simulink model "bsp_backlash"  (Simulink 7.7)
settings: Solver=ode45  StartTime=0.0  StopTime=10.0  MaxStep=0.1  RelTol=1e-3
StopFcn:
  | bsp_backlash_plot

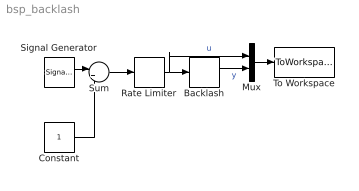
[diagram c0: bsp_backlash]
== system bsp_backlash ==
  Backlash : Backlash
  Constant : Constant
  Mux : Mux  Inputs=2
  Rate Limiter : RateLimiter
  Signal Generator : SignalGenerator  WaveForm=square  Frequency=0.4
  Sum : Sum  Inputs=|++
  To Workspace : ToWorkspace  VariableName=ausgabe  SampleTime=-1  SaveFormat=Array
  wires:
  Constant/1 -> Sum/2
  Signal Generator/1 -> Sum/1
  Rate Limiter/1 -> Backlash/1, Mux/1  "u"
  Mux/1 -> To Workspace/1
  Backlash/1 -> Mux/2  "y"
  Sum/1 -> Rate Limiter/1
